{attribute 'no_check'}
//Wrapper for available MDP_xxxx FBs of the lib, based on Beckhoff MDP - invalid values are reported via EventLogger 
//based on Tc2_MDP.lib - please see Beckhoff documentation for further information about Tc2_MDP.lib (IPC diagnostics)
FUNCTION_BLOCK MDP_Info EXTENDS FbBase
VAR_OUTPUT CONSTANT
	FNC_READ_ALL											:	INT := 0;
	FNC_READ_MOD_LIST										:	INT := 1;
	FNC_READ_MB												:	INT := 2;
	FNC_READ_CPU											:	INT := 3;
	FNC_READ_FAN											:	INT := 4;
	FNC_READ_SD												:	INT := 5;
	FNC_READ_RAID											:	INT := 6;
	FNC_READ_UPS											:	INT := 7;
END_VAR                 									
VAR_INPUT               									
	AmsNetId												: 	T_AmsNetId := '';	//AmsNetId as text
	Timeout													:	TIME := DEFAULT_ADS_TIMEOUT; //Ads timeout
	Fnc														:	INT (FNC_READ_ALL..FNC_READ_UPS) := FNC_READ_ALL; //select function to be read
(* Components *)            								
	ModList													:	MDP_ReadModulList;	//see content in FB
	MB														:	MDP_Mainboard;		//see content in FB
	CPU														:	MDP_CPU;			//see content in FB
	FAN														:	MDP_Fan;			//see content in FB
	SD														:	MDP_SiliconDrives;	//see content in FB
	RAID													:	MDP_RaidSimple;		//see content in FB
	UPS														:	MDP_UPS;			//see content in FB
END_VAR                     								
VAR_OUTPUT                  								
	TotalCycleTime											:	TIME;	//Cylce time to execute function block with mode read all        
	ErrorGrp												:	E_MDP_ErrGroup;
	ErrorFnc												:	STRING(15);
END_VAR
VAR
	MemFnc													:	INT;
	MemExecute												:	BOOL;
	MemErrorFnc												:	STRING(15);
	MemErrorid												:	UDINT;
	MemErrorGrp												:	E_MDP_ErrGroup;
	MemTimeStartCycle										:	TIME;
END_VAR

	(* Execute all available MDP_xxxxx fb 			*)
	(************************************************)

(* Sequence ********************************************)
	IF Execute
		AND state = 0
	THEN
		ReadAll(Execute	:= Execute);
	ELSIF state <> 0
	THEN
		ReadAll(Execute	:= Execute);
	END_IF

(*****************************************************************************)

METHOD PUBLIC readAll : BOOL //Return value = TRUE if busy;
VAR_INPUT
	Execute													:	BOOL;
END_VAR
	THIS^.Execute											:= Execute;

	IF Execute
		AND State = 0
	THEN
		MemFnc												:= Fnc;
		CASE Fnc OF                                     	
		FNC_READ_MOD_LIST:		state						:= 10;
		FNC_READ_MB:			state						:= 20;
		FNC_READ_CPU:			state						:= 30;
		FNC_READ_FAN:			state						:= 40;
		FNC_READ_SD:			state						:= 50;
		FNC_READ_RAID:	 		state						:= 60;
		FNC_READ_UPS:	 		state						:= 70;
		ELSE (* Read All *)
			MemFnc											:= FNC_READ_ALL;
			state											:= 10;
		END_CASE
		MemTimeStartCycle									:= TIME();
		Busy												:= TRUE;
		Done												:= FALSE;
		Error												:= FALSE;
		Errorid												:= 0;
		ErrorFnc											:= '';
		ErrorGrp											:= eMDP_Err_NoError;
		MemExecute											:= FALSE;
		MemErrorid											:= 0;
		MemErrorFnc											:= '';
		MemErrorGrp											:= eMDP_Err_NoError;
	ELSIF NOT Execute
		AND State = 99
	THEN
		Busy												:= FALSE;
		Done												:= FALSE;
		Error												:= FALSE;
		Errorid												:= 0;
		ErrorFnc											:= '';
		ErrorGrp											:= eMDP_Err_NoError;
		MemExecute											:= FALSE;
		MemErrorid											:= 0;
		MemErrorFnc											:= '';
		MemErrorGrp											:= eMDP_Err_NoError;
		ReadModList(FALSE);     						
		ReadMB(FALSE);
		ReadCPU(FALSE);
		ReadFAN(FALSE);
		ReadSD(FALSE);
		ReadRaid(FALSE);
	END_IF

	CASE state OF
	10:

		MemExecute											:= TRUE;
		ReadModList(MemExecute);
		IF NOT ModList.Busy
		THEN
			IF MemFnc = FNC_READ_ALL
			THEN
				IF Error AND MemErrorid = 0 
				THEN
					MemErrorId								:= Errorid; 
					MemErrorFnc 							:= CONCAT('ReadModList Fnc:',TO_STRING(FNC_READ_MOD_LIST)); 
					MemErrorGrp 							:= ErrorGrp;
				END_IF              						
				Busy										:= TRUE;
				Done										:= FALSE;
				Error										:= FALSE;
				Errorid										:= 0;
				ErrorGrp									:= eMDP_Err_NoError;
				state										:= 20;
			ELSE                    						
				state										:= 99;
			END_IF
		END_IF

	20:
		MemExecute											:= TRUE;
		ReadMB(MemExecute);
		IF NOT MB.Busy
		THEN
			IF MemFnc = FNC_READ_ALL
			THEN
				IF Error AND MemErrorid = 0 
				THEN
					MemErrorId								:= Errorid; 
					MemErrorFnc 							:= CONCAT('ReadMB Fnc: ',TO_STRING(FNC_READ_MB));  
					MemErrorGrp 							:= ErrorGrp;
				END_IF              						
				Busy										:= TRUE;
				Done										:= FALSE;
				Error										:= FALSE;
				Errorid										:= 0;
				ErrorGrp									:= eMDP_Err_NoError;
				state										:= 30;
			ELSE                    						
				state										:= 99;
			END_IF                  	
		END_IF

	30:
		MemExecute											:= TRUE;
		ReadCPU(MemExecute);
		IF NOT CPU.Busy
		THEN
			IF MemFnc = FNC_READ_ALL
			THEN
				IF Error AND MemErrorid = 0 THEN
					MemErrorId								:= Errorid; 
					MemErrorFnc 							:= CONCAT('ReadCPU Fnc: ',TO_STRING(FNC_READ_CPU));  
					MemErrorGrp 							:= ErrorGrp;
				END_IF              						
				Busy										:= TRUE;
				Done										:= FALSE;
				Error										:= FALSE;
				Errorid										:= 0;
				ErrorGrp									:= eMDP_Err_NoError;
				state										:= 40;
			ELSE                    						
				state										:= 99;
			END_IF
		END_IF

	40:
		MemExecute											:= TRUE;
		ReadFan(MemExecute);
		IF NOT Fan.Busy
		THEN
			IF MemFnc = FNC_READ_ALL
			THEN
				IF Error AND MemErrorid = 0 
				THEN
					MemErrorId								:= Errorid; 
					MemErrorFnc 							:= CONCAT('ReadFan Fnc: ',TO_STRING(FNC_READ_FAN));  
					MemErrorGrp 							:= ErrorGrp;
				END_IF              						
				Busy										:= TRUE;
				Done										:= FALSE;
				Error										:= FALSE;
				Errorid										:= 0;
				ErrorGrp									:= eMDP_Err_NoError;
				state										:= 50;
			ELSE                    						
				state										:= 99;
			END_IF
		END_IF

	50:
		MemExecute											:= TRUE;		
		ReadSD(MemExecute);
		
		IF NOT SD.Busy
		THEN
			IF MemFnc = FNC_READ_ALL
			THEN
				IF Error AND MemErrorid = 0 
				THEN				
					MemErrorId								:= Errorid; 
					MemErrorFnc 							:= CONCAT('ReadSD Fnc: ',TO_STRING(FNC_READ_SD)); 
					MemErrorGrp 							:= ErrorGrp;
				END_IF              						
				Busy										:= TRUE;
				Done										:= FALSE;
				Error										:= FALSE;
				Errorid										:= 0;
				ErrorGrp									:= eMDP_Err_NoError;
				state										:= 60;
			ELSE                    						
				state										:= 99;
			END_IF                  	
		END_IF

	60:
		MemExecute											:= TRUE;
		ReadRaid(MemExecute);
		IF NOT Raid.Busy
		THEN
			IF MemFnc = FNC_READ_ALL
			THEN
				IF Error AND MemErrorid = 0 
				THEN
					MemErrorId								:= Errorid; 
					MemErrorFnc 							:= CONCAT('ReadRaid Fnc: ',TO_STRING(FNC_READ_RAID));
					MemErrorGrp 							:= ErrorGrp;
				END_IF              						
				Busy										:= TRUE;
				Done										:= FALSE;
				Error										:= FALSE;
				Errorid										:= 0;
				ErrorGrp									:= eMDP_Err_NoError;
				state										:= 70;
			ELSE                    						
				state										:= 99;
			END_IF
		END_IF

	70:
		MemExecute											:= TRUE;
		ReadUPS(MemExecute);
		IF NOT UPS.Busy
		THEN
			IF TRUE
			THEN
				IF Error AND MemErrorid = 0 
				THEN
					MemErrorId								:= Errorid; 
					MemErrorFnc 							:= CONCAT('ReadUPS Fnc: ',TO_STRING(FNC_READ_UPS));
					MemErrorGrp 							:= ErrorGrp;
				END_IF
				Busy										:= FALSE;
				Done										:= MemErrorId = 0;
				Error										:= MemErrorId <> 0;
				Errorid										:= MemErrorid;
				ErrorFnc									:= MemErrorFnc;
				ErrorGrp									:= MemErrorGrp;
				state										:= 99;
			ELSE                    						
				state										:= 99;
			END_IF
		END_IF

	99:;
	
	END_CASE

	IF state = 99
	THEN
		TotalCycleTime	 									:= TIME() - MemTimeStartCycle;
		IF NOT Execute
		THEN
			state											:= 0;
			ReadModList(FALSE);         					
			ReadMB(FALSE);              					
			ReadCPU(FALSE);             					
			ReadFAN(FALSE);             					
			ReadSD(FALSE);              					
			ReadRaid(FALSE);            					
			ReadUPS(FALSE);             	
		END_IF                          	
	END_IF                              	
	                                    	
	ReadAll													:= Busy;

(***********************************************************************************)
END_METHOD

METHOD PUBLIC readCPU : BOOL //Return value = TRUE if busy
VAR_INPUT
	Execute													:	BOOL;
END_VAR
THIS^.Execute												:= Execute;

CPU(
	Execute				:= MemExecute OR Execute,
	AmsNetId			:= AmsNetId,
	Timeout				:= Timeout,
	MIN_CPU				=> ,
	MAX_CPU				=> ,
	Busy				=> Busy,
	Done				=> Done,
	Error				=> Error,
	ErrorId				=> Errorid,
	ErrorGrp 			=> ErrorGrp,
	Frequency			=> ,
	Usage				=> ,
	Temperature			=> ,
	AverageFrequency	=> ,
	AverageUsage		=> ,
	AverageTemperature	=> ,
	Count				=> );

MemExecute 													:= FALSE;
	        												
ReadCPU														:= Busy;
END_METHOD

METHOD PUBLIC readFan : BOOL //Return value = TRUE if busy
VAR_INPUT
	Execute													:	BOOL;
END_VAR
THIS^.Execute												:= Execute;

FAN(
	Execute		:= MemExecute OR Execute,
	AmsNetId	:= AmsNetid,
	Timeout		:= Timeout,
	MIN_FAN		=> ,
	MAX_FAN		=> ,
	Busy		=> Busy,
	Done		=> Done,
	Error		=> Error,
	ErrorId		=> ErrorId,
	ErrorGrp 	=> ErrorGrp,
	Speed		=> ,
	Count		=> );

MemExecute 													:= FALSE;
           												
ReadFan														:= Busy;
END_METHOD

METHOD PUBLIC readMB : BOOL //Return value = TRUE if busy
VAR_INPUT
	Execute													:	BOOL;
END_VAR
THIS^.Execute												:= Execute;

MB(
	Execute			:= MemExecute OR Execute,
	AmsNetId		:= AmsNetId,
	Timeout			:= Timeout,
	MIN_VOLTAGE		=> ,
	MAX_VOLTAGE		=> ,
	Busy			=> Busy,
	Done			=> Done,
	Error			=> Error,
	ErrorId			=> ErrorId,
	ErrorGrp		=> Errorgrp,
	MB_Type			=> ,
	SerielNo		=> ,
	ProdDate		=> ,
	BootCount		=> ,
	OpTime			=> ,
	MinBoardTemp	=> ,
	MaxBoardTemp	=> ,
	MinInputVolt	=> ,
	MaxInputVolt	=> ,
	MB_Temp			=> ,
	VoltLocation	=> ,
	VoltageValue	=> ,
	VoltageNominal	=> ,
	VoltCount		=> );

MemExecute 													:= FALSE;
            												
ReadMB														:= Busy;
END_METHOD

METHOD PUBLIC readModList : BOOL //Return value = TRUE if busy
VAR_INPUT
	Execute													:	BOOL;
END_VAR
THIS^.Execute												:= Execute;

ModList(
	Execute		:= MemExecute OR Execute,
	AmsNetId	:= AmsNetId,
	Timeout		:= Timeout,
	Busy		=> Busy,
	Done		=> done,
	Error		=> Error,
	ErrorId		=> ErrorId,
	ErrorGrp 	=> ErrorGrp );

MemExecute 													:= FALSE;
            												
ReadModList													:= Busy;
END_METHOD

METHOD PUBLIC readRaid : BOOL //Return value = TRUE if busy
VAR_INPUT
	Execute													: BOOL;
END_VAR
THIS^.Execute												:= Execute;

RAID(
	Execute			:= Execute OR MemExecute,
	AmsNetId		:= AmsNetId,
	Timeout			:= timeout,
	MIN_DRIVE		=> ,
	MAX_DRIVE		=> ,
	Busy			=> Busy,
	Done			=> done,
	Error			=> Error,
	ErrorId			=> ErrorId,
	ErrorGrp 		=> ErrorGrp,
	CntrState		=> ,
	CntrOfflReason	=> ,
	SetType			=> ,
	SetState		=> ,
	SetInfo			=> ,
	CountDrives		=> ,
	DriveSTATE		=> ,
	CountRAIDSets	=> );

MemExecute 													:= FALSE;
                											
ReadRaid													:= Busy;
END_METHOD

METHOD PUBLIC readSD : BOOL //Return value = TRUE if busy
VAR_INPUT
	Execute		:	BOOL;
END_VAR
THIS^.Execute												:= Execute;

SD(
	Execute			:= MemExecute OR Execute,
	AmsNetId		:= AmsNetid,
	Timeout			:= timeout,
	MIN_DRIVES		=> ,
	MAX_DRIVES		=> ,
	Busy			=> Busy,
	Done			=> Done,
	Error			=> Error,
	ErrorId			=> Errorid,
	ErrorGrp 		=> ErrorGrp,
	TotEraseCounts	=> ,
	Usage			=> ,
	NoOfSpares		=> ,
	SparedUsed		=> ,
	Count			=> );

MemExecute	 												:= FALSE;
                											
ReadSD														:= Busy;
END_METHOD

METHOD PUBLIC readUPS : Bool //Return value = TRUE if busy
VAR_INPUT
	Execute		:	BOOL;
END_VAR
THIS^.Execute												:= Execute;

UPS(
	Execute					:= MemExecute OR Execute,
	AmsNetId				:= AmsNetid,
	Timeout					:= timeout,
	Busy					=> Busy,
	Done					=> Done,
	Error					=> Error,
	ErrorId					=> Errorid,
	ErrorGrp				=> ErrorGrp,
	Model					=> ,
	VendorName				=> ,
	PowerStatus				=> ,
	ComStatus				=> ,
	BatteryStatus			=> ,
	BatteryCapacity			=> ,
	BatteryRuntime			=> ,
	PersPowerFailCounter	=> ,
	PowerFailCounter		=> ,
	FanError				=> ,
	NoBattery				=> );

MemExecute 													:= FALSE;
ReadUPS														:= Busy;
END_METHOD

END_FUNCTION_BLOCK
